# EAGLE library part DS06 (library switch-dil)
DIL/CODE SWITCH
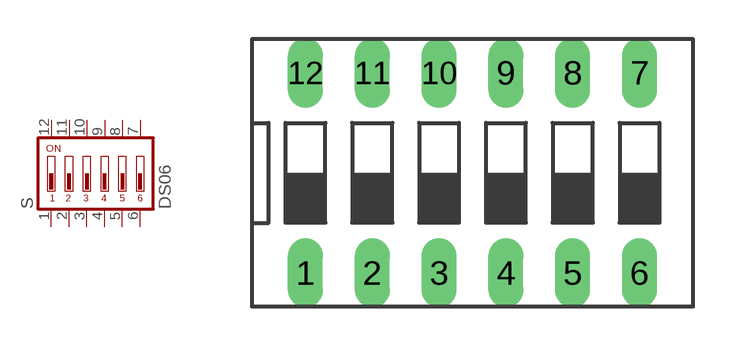
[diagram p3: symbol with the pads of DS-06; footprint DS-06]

Designator prefix S

## DS06 (MPN: MCDS06; OC_FARNELL: 9471588; OC_NEWARK: 26M1105)  [DS-06]
1  1  pas
2  2  pas
3  3  pas
4  4  pas
5  5  pas
6  6  pas
7  7  pas
8  8  pas
9  9  pas
10  10  pas
11  11  pas
12  12  pas

## Footprint DS-06 (pad centres in mm)
DIL/CODE SWITCH Mors distributor Buerklin, 17G558
drill 0.813 long: 1 -6.35,-3.81; 2 -3.81,-3.81; 3 -1.27,-3.81; 4 1.27,-3.81; 5 3.81,-3.81; 6 6.35,-3.81; 7 6.35,3.81; 8 3.81,3.81; 9 1.27,3.81; 10 -1.27,3.81; 11 -3.81,3.81; 12 -6.35,3.81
